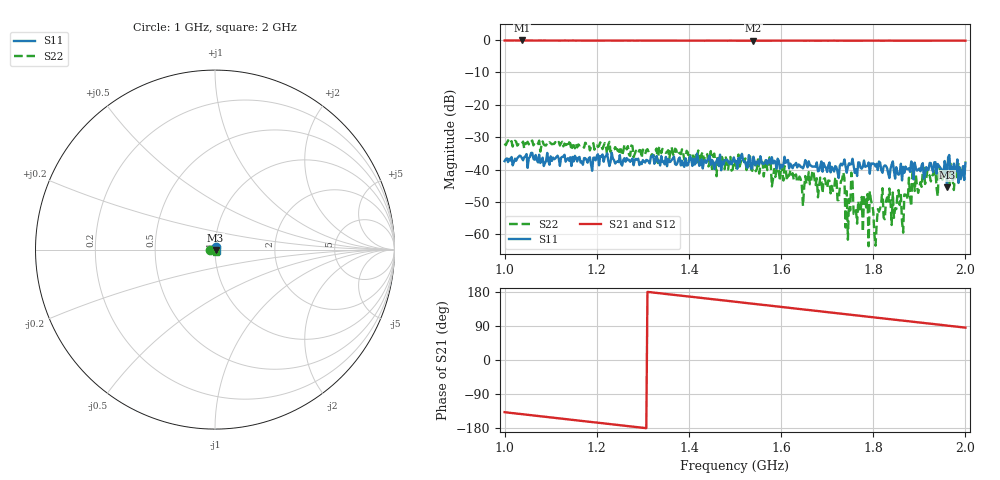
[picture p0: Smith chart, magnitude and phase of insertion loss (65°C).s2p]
!Agilent Technologies,E8363C,MY43030407,A.09.42.15
!Agilent E8363C: A.09.42.15
!Date: Friday, September 05, 2025 18:27:19
!Correction: S11(Full 2 Port(1,2))
!S21(Full 2 Port(1,2))
!S12(Full 2 Port(1,2))
!S22(Full 2 Port(1,2))
!S2P File: Measurements: S11, S21, S12, S22:
# Hz S  dB  R 50
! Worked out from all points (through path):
!   401 points, 1 GHz to 2 GHz, reference 50 ohm
!   highest |S21| = -0.11 dB at 1.038 GHz (marker M1); lowest = -0.2 dB at 1.54 GHz (marker M2)
!   group delay of S21, straight-line fit = 380 ps
!   lowest |S11| = -45.4 dB at 1.96 GHz (marker M3), VSWR 1.01, Z = 50.4 - j0.404 ohm
!   |S11| at or under -10 dB: start of sweep to end of sweep
!   |S22| runs from -63.6 to -31.0 dB; largest |S21 - S12| = 0.0068
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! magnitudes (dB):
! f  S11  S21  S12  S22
! 1 GHz  -37.4  -0.1  -0.1  -32.0
! 1.038 GHz  -36.4  -0.1  -0.1  -32.0
! 1.167 GHz  -37.5  -0.2  -0.2  -32.5
! 1.335 GHz  -37.2  -0.2  -0.2  -33.3
! 1.5 GHz  -37.6  -0.2  -0.2  -38.4
! 1.54 GHz  -36.0  -0.2  -0.2  -38.4
! 1.573 GHz  -37.1  -0.2  -0.2  -38.5
! 1.65 GHz  -38.7  -0.2  -0.2  -45.6
! 1.667 GHz  -39.1  -0.2  -0.2  -40.9
! 1.728 GHz  -38.8  -0.2  -0.2  -45.5
! 1.732 GHz  -38.7  -0.2  -0.2  -43.0
! 1.745 GHz  -39.1  -0.2  -0.2  -61.7
! 1.752 GHz  -38.3  -0.2  -0.2  -40.9
! 1.762 GHz  -39.9  -0.2  -0.2  -52.5
! 1.798 GHz  -38.3  -0.2  -0.2  -50.8
! 1.805 GHz  -39.0  -0.2  -0.2  -63.5
! 1.815 GHz  -37.9  -0.2  -0.2  -52.0
! 1.835 GHz  -42.6  -0.1  -0.2  -45.8
! 1.863 GHz  -43.3  -0.2  -0.2  -56.1
! 1.89 GHz  -37.9  -0.2  -0.2  -46.6
! 1.96 GHz  -45.4  -0.2  -0.2  -40.5
! 2 GHz  -38.0  -0.2  -0.2  -37.5
